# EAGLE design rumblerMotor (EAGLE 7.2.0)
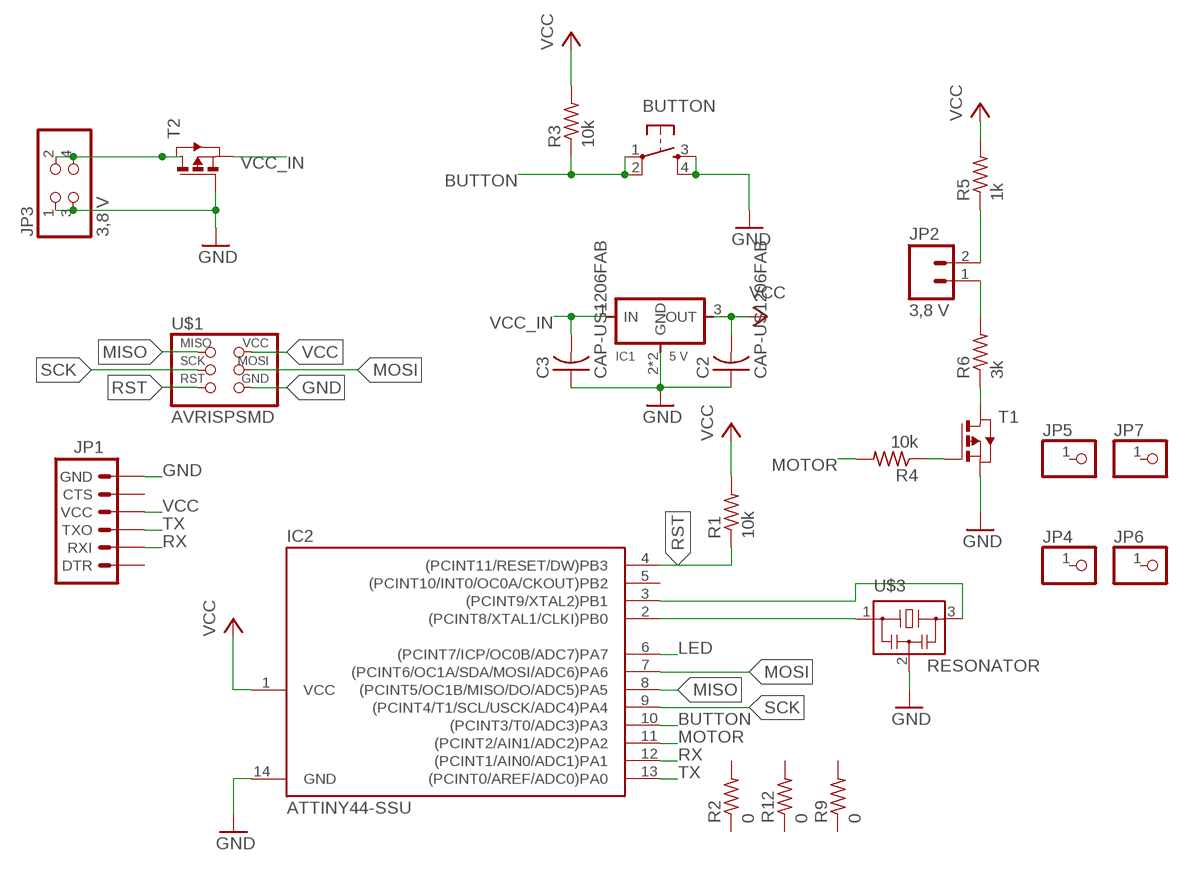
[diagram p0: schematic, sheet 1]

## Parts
BUTTON  6MM_SWITCH6MM_SWITCH  [6MM_SWITCH]
C2  CAP-US1206FAB  [C1206FAB]
C3  CAP-US1206FAB  [C1206FAB]
IC1  5 V  REGULATORSOT223  [SOT223]
IC2  ATTINY44-SSU  [SOIC14]
JP1  ARDUINO_SERIAL_PROGRAMSMD  [1X06-SMD]
JP2  3,8 V  M023.5MM_LOCK  [SCREWTERMINAL-3.5MM-2_LOCK]
JP3  3,8 V  PINHD-2X2-SMD  [2X02SMD]
JP4  PINHD-1X1CB  [1X01-CLEANBIG]
JP5  PINHD-1X1CB  [1X01-CLEANBIG]
JP6  PINHD-1X1CB  [1X01-CLEANBIG]
JP7  PINHD-1X1CB  [1X01-CLEANBIG]
R1  10k  RES-US1206FAB  [R1206FAB]
R2  0  RES-US1206FAB  [R1206FAB]
R3  10k  RES-US1206FAB  [R1206FAB]
R4  10k  RES-US1206FAB  [R1206FAB]
R5  1k  RES-US1206FAB  [R1206FAB]
R6  3k  RES-US1206FAB  [R1206FAB]
R9  0  RES-US1206FAB  [R1206FAB]
R12  0  RES-US1206FAB  [R1206FAB]
T1  PMOSFETSOT23  [SOT-23]
T2  PMOSFETSOT23  [SOT-23]
U$1  AVRISPSMD  [2X03SMD]
U$3  RESONATOR  [EFOBM]

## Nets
BUTTON: BUTTON.1(P) BUTTON.2(P1) IC2.10((PCINT3/T0/ADC3)PA3) R3.1
GND: BUTTON.3(S) BUTTON.4(S1) C2.1 C3.1 IC1.2(GND) IC1.4(GND) IC2.14(GND) JP1.6(GND) JP3.1 JP3.3 T1.2(S) T2.3(G) U$1.6(GND) U$3.2
LED: IC2.6((PCINT7/ICP/OC0B/ADC7)PA7)
MISO: IC2.8((PCINT5/OC1B/MISO/DO/ADC5)PA5) U$1.1(MISO)
MOSI: IC2.7((PCINT6/OC1A/SDA/MOSI/ADC6)PA6) U$1.4(MOSI)
MOTOR: IC2.11((PCINT2/AIN1/ADC2)PA2) R4.2
N$1: JP2.2 R5.1
N$3: IC2.2((PCINT8/XTAL1/CLKI)PB0) U$3.1
N$4: IC2.3((PCINT9/XTAL2)PB1) U$3.3
N$5: JP2.1 R6.2
N$6: R6.1 T1.1(D)
N$7: JP3.2 JP3.4 T2.1(D)
N$8: R4.1 T1.3(G)
RST: IC2.4((PCINT11/RESET/DW)PB3) R1.1 U$1.5(RST)
RX: IC2.12((PCINT1/AIN0/ADC1)PA1) JP1.2(RXI)
SCK: IC2.9((PCINT4/T1/SCL/USCK/ADC4)PA4) U$1.3(SCK)
TX: IC2.13((PCINT0/AREF/ADC0)PA0) JP1.3(TXO)
VCC: C2.2 IC1.3(OUT) IC2.1(VCC) JP1.4(VCC) R1.2 R3.2 R5.2 U$1.2(VCC)
VCC_IN: C3.2 IC1.1(IN) T2.2(S)
Unconnected: IC2.5((PCINT10/INT0/OC0A/CKOUT)PB2) JP1.1(DTR) JP1.5(CTS) JP4.1 JP5.1 JP6.1 JP7.1 R2.1 R2.2 R9.1 R9.2 R12.1 R12.2

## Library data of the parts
BUTTON = 01_fab:6MM_SWITCH: OMRON SWITCH
C2 C3 = 01_fab:CAP-US
IC1 = 01_fab:REGULATOR
IC2 = 01_fab:ATTINY44
JP1 = SparkFun-Connectors:ARDUINO_SERIAL_PROGRAM: FTDI connector footprints
JP2 = SparkFun-Connectors:M02: Standard 2-pin 0.1" header. Use with; PROD_ID: CONN-08399
JP3 = fab:PINHD-2X2-SMD
JP4-JP7 = adafruit:PINHD-1X1: Pin header 1x1 for 0.1" spacing
R1-R6 R9 R12 = 01_fab:RES-US: Resistor (US Symbol)
T1 T2 = 01_fab:PMOSFET: MOS FET
U$1 = fab:AVRISP
U$3 = 01_fab:RESONATOR

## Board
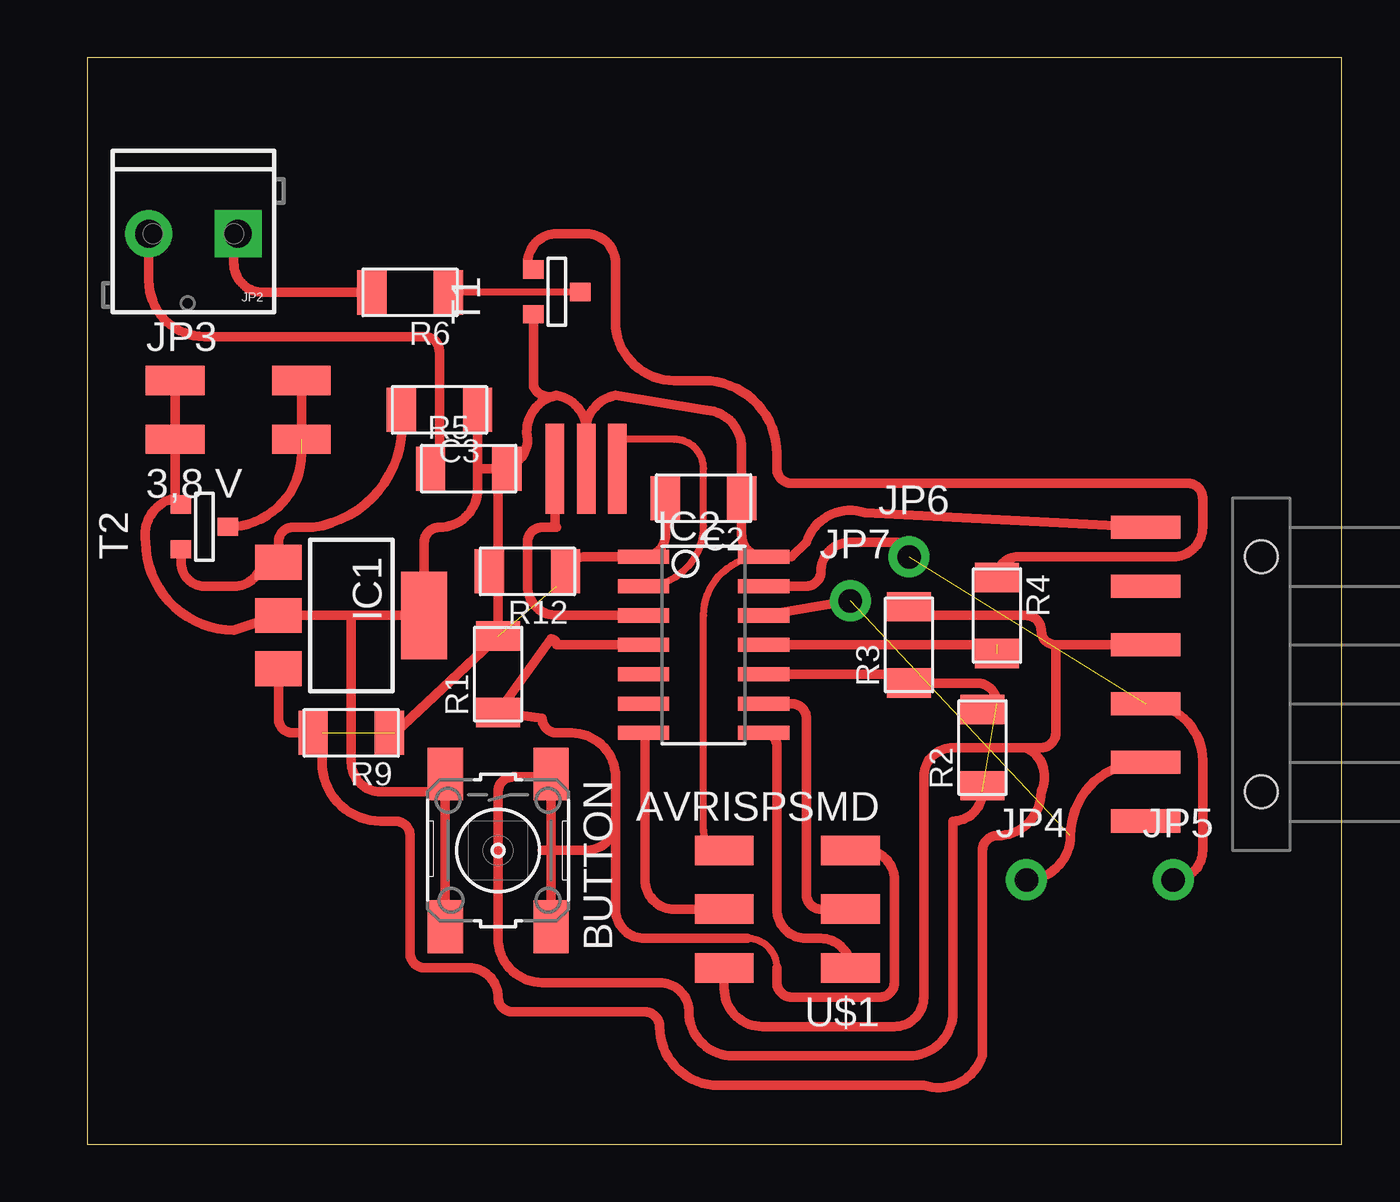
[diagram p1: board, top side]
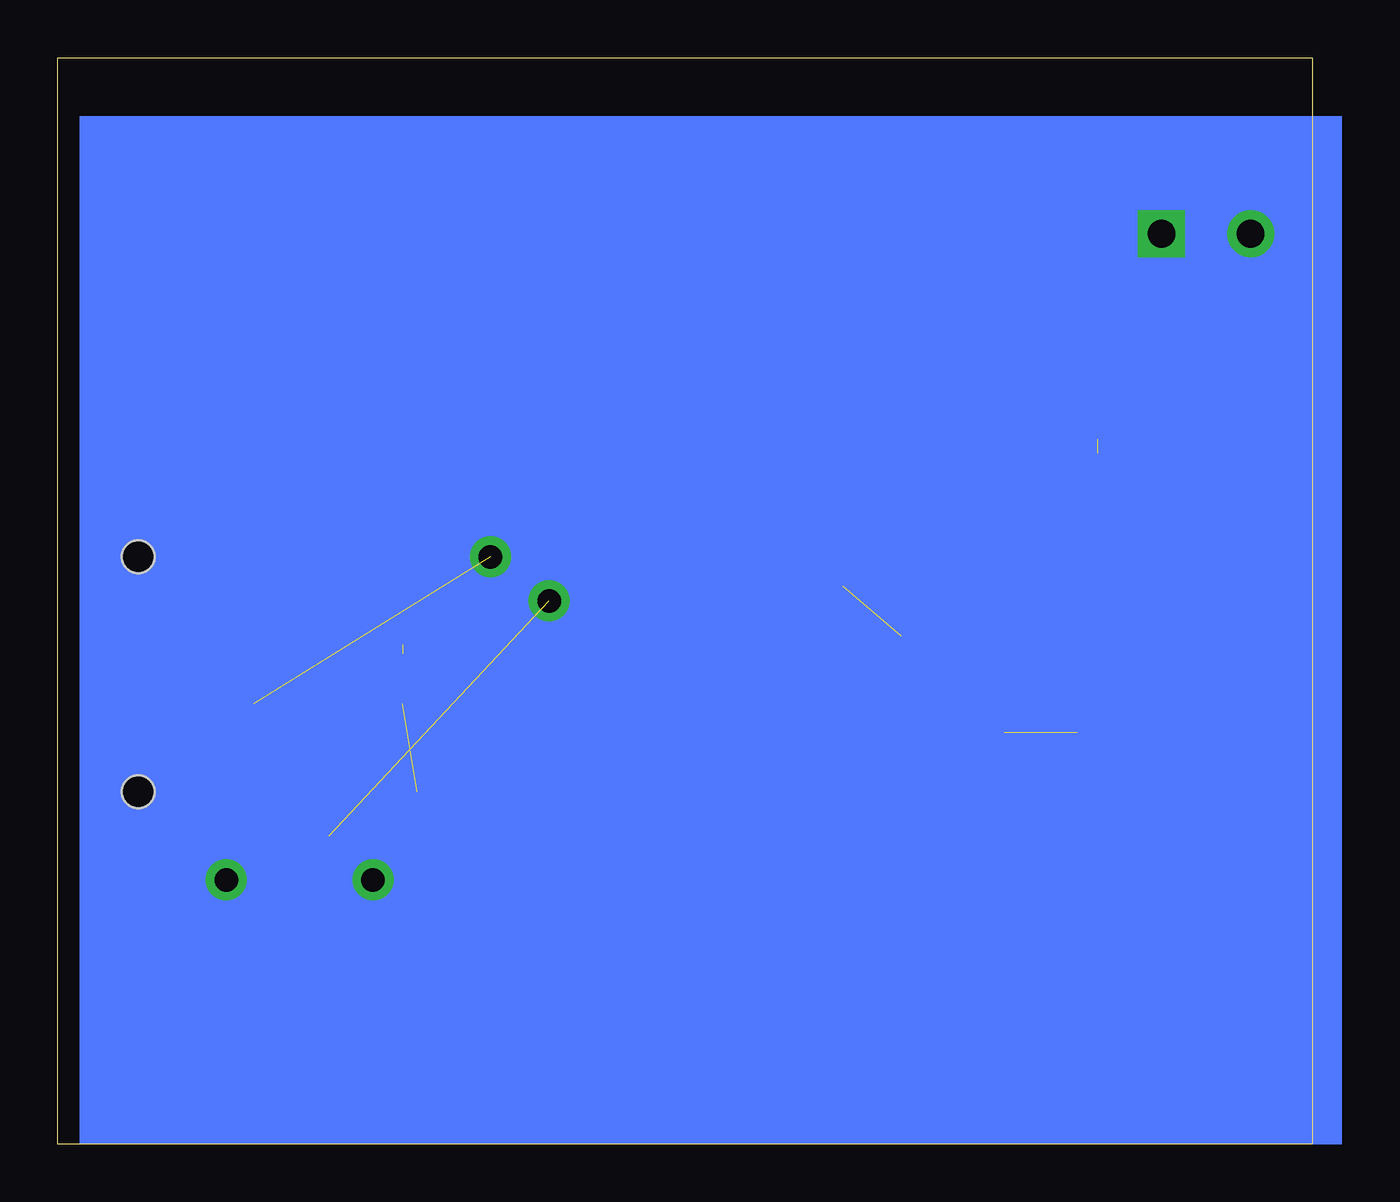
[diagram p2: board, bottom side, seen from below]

Size 54.28 x 46.98 mm. Coordinates in mm from the lower left corner, seen from the top.
Outline: 0,0 54.28,0 54.28,46.98 0,46.98 0,0
Copper layers (1*16): Top 0.035mm / dielectric 1.5mm / Bottom 0.035mm
Design rules "fabmodule": minimum track width 10mil, minimum drill 0.4mm, track to track 0.42mm, track to pad 0.42mm, pad to pad 0.42mm, via to via 0.42mm, smd to smd 0.42mm, copper to edge 40mil, drill to drill 0.8mm, minimum pad ring 10mil, minimum via ring 8mil, stop-mask expansion 4mil, vias tented up to drill 0mil, thermal gap 10mil

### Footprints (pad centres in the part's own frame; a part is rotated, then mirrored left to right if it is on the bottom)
6MM_SWITCH = smd 2.286 x 1.524: 1 -3.302,2.286; 2 3.302,2.286; 3 -3.302,-2.286; 4 3.302,-2.286
C1206FAB = smd 1.27 x 1.905: 1 -1.651,0; 2 1.651,0
SOT223 = smd 1.5 x 2: 1 -2.3,-3.15; 2 0,-3.15; 3 2.3,-3.15 | smd 3.8 x 2: 4 0,3.15
SOIC14 = smd 0.61 x 2.21: 1 -3.81,-2.603; 2 -2.54,-2.603; 3 -1.27,-2.603; 4 0,-2.603; 5 1.27,-2.603; 6 2.54,-2.603; 7 3.81,-2.603; 8 3.81,2.603; 9 2.54,2.603; 10 1.27,2.603; 11 0,2.603; 12 -1.27,2.603; 13 -2.54,2.603; 14 -3.81,2.603
1X06-SMD = smd 1 x 3: 1 -6.35,5; 2 -3.81,5; 3 -1.27,5; 4 1.27,5; 5 3.81,5; 6 6.35,5 | hole 1.4: -5.08,0; 5.08,0
SCREWTERMINAL-3.5MM-2_LOCK = drill 1.2 pad 2.032 square: 1 -0.178,0 | drill 1.2 pad 2.032: 2 3.678,0
2X02SMD = smd 2.54 x 1.27: 1 -2.54,1.27; 2 2.92,1.27; 3 -2.54,-1.27; 4 2.92,-1.27
1X01-CLEANBIG = drill 1.016 pad 1.778: 1 0,0
R1206FAB = smd 1.27 x 1.905: 1 -1.651,0; 2 1.651,0
SOT-23 = smd 0.787 x 0.889: 1 0.025,-1.016; 2 -0.94,1.016; 3 0.991,1.016
2X03SMD = smd 2.54 x 1.27: 1 -2.54,2.54; 2 2.92,2.54; 3 -2.54,0; 4 2.92,0; 5 -2.54,-2.54; 6 2.92,-2.54
EFOBM = smd 0.8 x 3.9: 1 -1.35,0; 2 0,0; 3 1.35,0

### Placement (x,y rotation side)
BUTTON  17.78,12.7 270 top
C2  26.67,27.94 180 top
C3  15.24,31.75 180 top
IC1  11.43,22.86 270 top
IC2  26.67,21.59 270 top
JP1  50.8,20.32 90 top
JP2  6.35,39.37 180 top
JP3  6.35,31.75 0 top
JP4  40.64,11.43 0 top
JP5  46.99,11.43 0 top
JP6  35.56,25.4 0 top
JP7  33.02,23.49 0 top
R1  17.78,20.32 90 top
R2  38.73,17.15 90 top
R3  35.56,21.59 90 top
R4  39.37,22.86 270 top
R5  16.51,29.21 0 top
R6  13.97,36.83 180 top
R9  11.43,17.78 180 top
R12  19.05,24.77 180 top
T1  20.32,36.83 90 top
T2  5.08,26.67 90 top
U$1  30.48,10.16 180 top
U$3  21.59,29.21 180 top

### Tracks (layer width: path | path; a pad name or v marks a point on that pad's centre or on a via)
BUTTON  (1 unrouted)
  Top 0.406: BUTTON.2 BUTTON.1 arc-90 19.94,15.87 18.41,15.87 arc90 17.78,15.24 17.78,8.89 arc90 19.69,6.98 24.77,6.98 arc-90 26.03,5.71 arc90 27.94,3.81 35.56,3.81 arc90 37.46,5.71 37.46,13.97 arc90 38.73,15.24 | 39.37,19.05 arc90 38.48,19.94 R3.1 35.18,20.32 IC2.10
GND
  Top 0.305: U$1.6 arc-90 26.67,13.59 26.67,22.86 arc-90 29.21,25.4
  Top 0.406: IC2.14 arc-90 28.32,26.35 C2.1 28.32,30.1 arc90 26.67,31.75 22.86,32.39 arc90 21.59,30.48 | U$3.2 21.59,30.48 | 21.59,30.48 arc90 20.32,32.39 | 20.32,32.39 arc90 19.05,30.48 arc-90 17.78,29.21 16.89,29.21 | 29.21,25.4 IC2.14 | C3.1 16.89,29.21 | 16.89,29.21 16.89,28.32 arc-90 15.24,26.67 arc90 14.58,26.01 IC1.4 11.43,22.86 | BUTTON.4 BUTTON.3 arc-90 14.73,15.24 12.7,15.24 arc-90 11.43,16.51 11.43,22.86 | T1.2 19.3,32.77 arc90 20.32,32.39 | IC2.14 30.48,25.4 31.12,26.03 arc-90 33.66,27.3 JP1.6 | 11.43,22.86 IC1.2 6.35,22.23 arc-90 2.54,26.03 arc-90 3.81,27.94 | JP3.1 JP3.3 3.81,27.94 | 3.81,27.94 3.81,27.91 arc90 T2.3
MISO
  Top 0.406: U$1.1 arc90 31.75,8.89 31.12,8.89 arc-90 29.84,10.16 29.84,17.21 arc90 IC2.8
MOSI
  Top 0.406: U$1.4 25.4,10.16 arc-90 24.13,11.43 24.13,17.72 arc90 IC2.7
MOTOR  (1 unrouted)
  Top 0.406: IC2.11 39.37,21.59
N$1
  Top 0.406: JP2.2 2.67,37.33 arc90 5.08,34.93 14.6,34.93 arc-90 15.24,34.29 15.24,29.59 arc-90 R5.1
N$3
  Top 0.305: IC2.2 arc90 26.67,26.73 26.67,29.21 arc90 25.4,30.48 22.86,30.48 arc-90 22.94,30.4 U$3.1
N$4
  Top 0.406: U$3.3 20.24,26.75 arc90 20.32,26.67 19.69,26.67 arc90 19.05,26.03 19.05,24.13 arc90 20.32,22.86 IC2.3
N$5
  Top 0.406: R6.2 7.62,36.83 arc-90 6.35,38.1 6.35,39.19 arc-90 JP2.1
N$6
  Top 0.305: 15.65,36.86 T1.1
  Top 0.406: 15.65,36.86 arc90 R6.1
N$7  (1 unrouted)
  Top 0.406: JP3.2 9.27,29.87 arc-90 T2.1
N$8
  Top 0.406: T1.3 arc-90 19.05,38.08 19.05,38.1 arc-90 20.32,39.37 21.59,39.37 arc-90 22.86,38.1 22.86,35.56 arc90 25.4,33.02 26.67,33.02 arc-90 29.84,29.84 29.84,29.21 arc90 30.48,28.58 47.62,28.58 arc-90 48.26,27.94 48.26,26.67 arc-90 46.99,25.4 40.26,25.4 arc90 R4.1
RST
  Top 0.305: 29.84,7.62 arc90 28.57,8.89
  Top 0.406: U$1.5 33.66,12.7 arc-90 34.93,11.43 34.93,6.98 arc-90 34.29,6.35 30.48,6.35 arc-90 29.84,6.98 29.84,7.62 | IC2.4 20.32,21.59 arc90 20.07,21.84 R1.1 19.69,18.41 arc90 20.32,17.78 20.95,17.78 arc-90 22.86,15.87 22.86,13.97 | 28.57,8.89 24.13,8.89 arc-90 22.86,10.16 22.86,13.97 | 19.69,12.7 21.59,12.7 arc90 22.86,13.97
RX  (1 unrouted)
  Top 0.406: 46.99,16.51 JP1.2 45.72,16.51 arc90 42.54,13.33 arc-90 40.64,11.43 | IC2.12 33.02,23.49
SCK
  Top 0.406: IC2.9 30.48,19.05 arc-90 31.12,18.41 31.12,10.79 arc90 31.75,10.16 U$1.3
TX  (1 unrouted)
  Top 0.406: JP1.3 arc-90 48.26,16.59 48.26,12.7 arc-90 46.99,11.43 | IC2.13 31.12,24.13 arc90 31.75,24.77 arc-90 33.02,26.03 34.93,26.03 arc-90 35.56,25.4
VCC  (2 unrouted)
  Top 0.406: C2.2 25.02,26.35 arc-90 IC2.1 21.59,25.4 arc90 20.32,24.13 | U$1.2 27.56,6.73 arc90 29.21,5.08 34.93,5.08 arc90 36.2,6.35 36.2,15.87 arc-90 37.46,17.15 40.64,17.15 | 41.27,22.23 arc90 40.64,22.86 | 41.27,22.23 arc90 40.64,22.86 | 40.64,22.86 35.94,22.86 arc-90 R3.2 | 41.27,22.23 arc90 41.91,21.59 | 41.91,21.59 JP1.4 | R1.2 17.78,28.83 arc-90 R5.2 | IC1.3 8.28,18.39 arc90 8.89,17.78 10.16,17.78 10.16,16.51 arc90 12.7,13.97 13.34,13.97 arc-90 13.97,13.33 13.97,8.26 arc90 14.6,7.62 16.51,7.62 arc-90 17.78,6.35 arc90 18.41,5.71 24.13,5.71 arc-90 24.77,5.08 arc90 27.3,2.54 36.2,2.54 arc90 38.73,3.81 38.73,12.7 arc-90 39.37,13.33 arc90 41.27,15.24 arc90 40.64,17.15 | R1.2 16.89,21.97 | 40.64,17.15 41.27,17.15 arc90 41.91,17.78 41.91,21.59 | R1.2 17.78,21.59 | 13.34,17.78 R1.2
VCC_IN
  Top 0.406: C3.2 arc-90 9.78,26.67 8.89,26.67 arc90 8.28,26.06 IC1.1 arc90 8.04,25.4 7.62,25.4 arc-90 6.35,24.13 5.08,24.13 arc-90 4.06,25.15 T2.2
(copper drawn outside any net)
  shapes: Bottom area x1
